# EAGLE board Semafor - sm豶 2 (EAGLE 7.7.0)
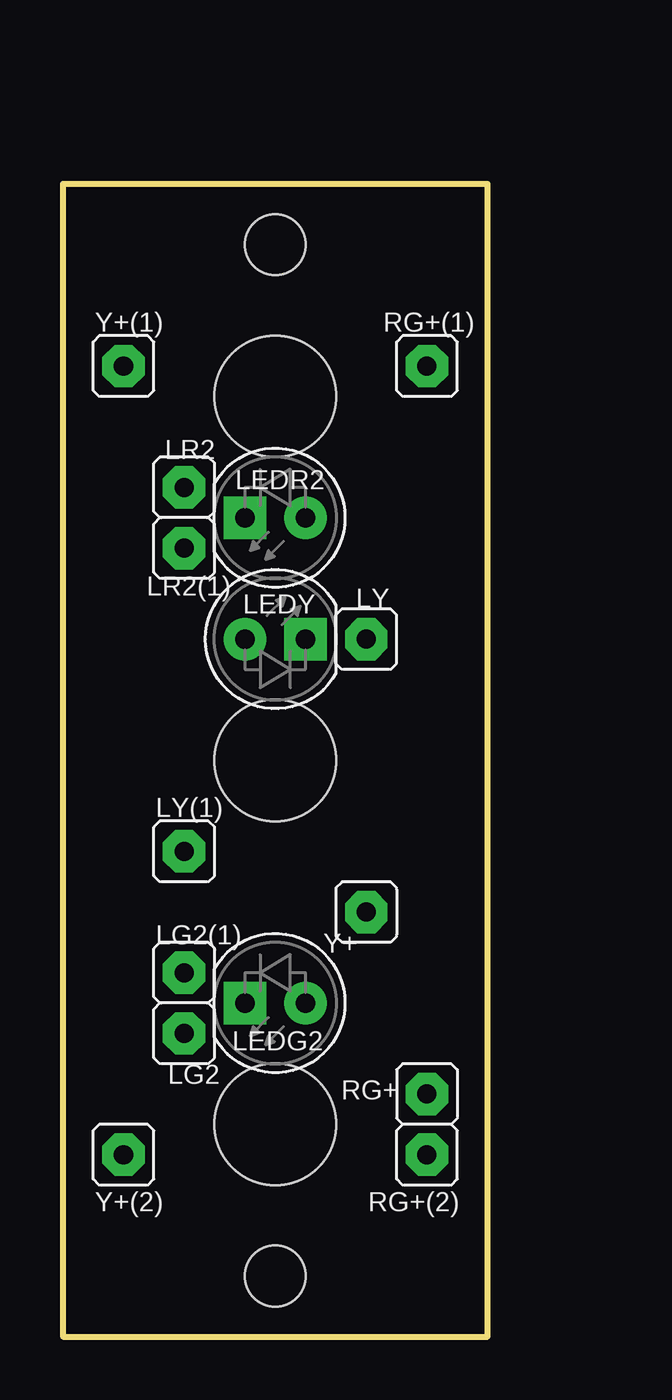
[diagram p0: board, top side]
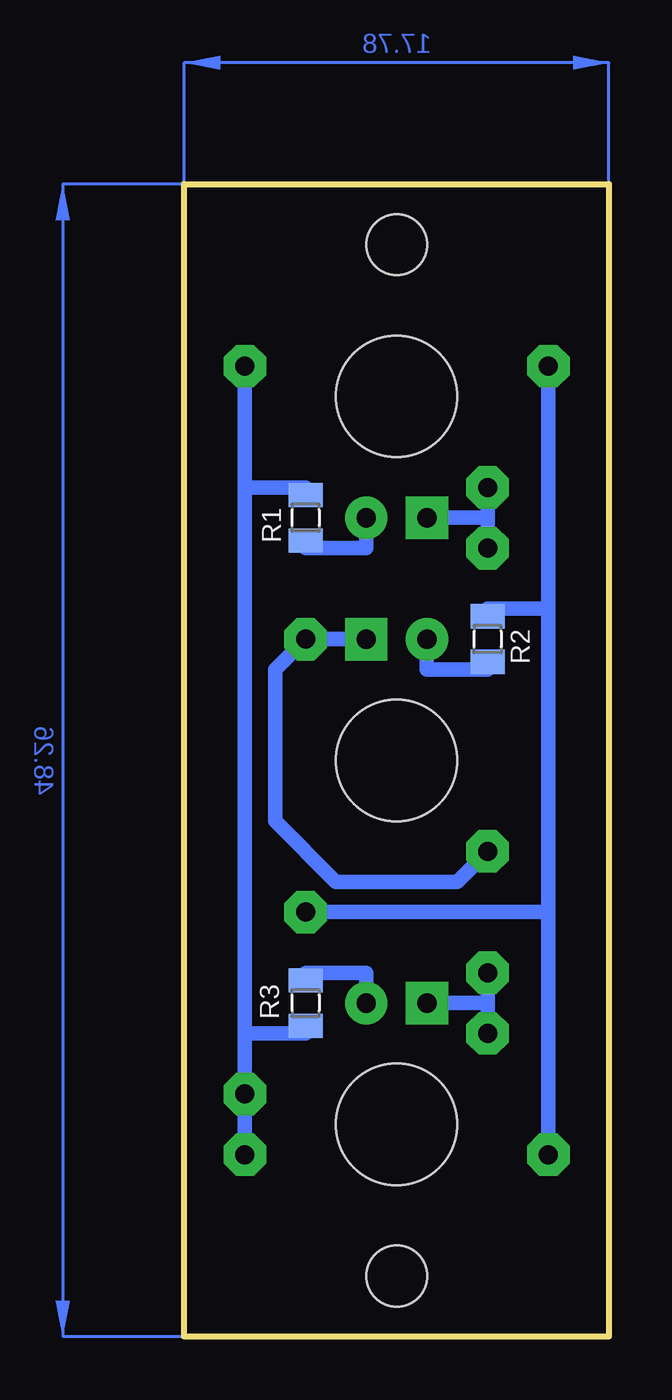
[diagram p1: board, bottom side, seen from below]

Size 17.78 x 48.26 mm. Coordinates in mm from the lower left corner, seen from the top.
Outline: 0,0 17.78,0 17.78,48.26 0,48.26 0,0
Copper layers (1*16): Top 0.035mm / dielectric 1.5mm / Bottom 0.035mm
Design rules "default": minimum track width 10mil, minimum drill 24mil, track to track 8mil, track to pad 8mil, pad to pad 8mil, via to via 8mil, smd to smd 8mil, copper to edge 40mil, drill to drill 8mil, minimum pad ring 10mil, minimum via ring 8mil, stop-mask expansion 4mil, vias tented up to drill 0mil, thermal gap 10mil
Holes 5.08 mm at 8.89,39.37 8.89,24.13 8.89,8.89
Holes 2.54 mm at 8.89,2.54 8.89,45.72

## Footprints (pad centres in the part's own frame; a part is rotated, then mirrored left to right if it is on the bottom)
LED_5 = drill 0.813 pad 1.778: A -1.27,0 | drill 0.813 pad 1.778 square: K 1.27,0
S1G1_JUM = drill 0.8 pad 1.778 octagon: 1 0,0
0805 = smd 1.016 x 1.422: 1 -0.953,0; 2 0.953,0

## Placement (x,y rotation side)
LEDG2  [LED_5]  8.89,13.97 180 top
LEDR2  [LED_5]  8.89,34.29 180 top
LEDY  [LED_5]  8.89,29.21 0 top
LG2  [S1G1_JUM]  5.08,12.7 270 top
LG2(1)  [S1G1_JUM]  5.08,15.24 270 top
LR2  [S1G1_JUM]  5.08,35.56 270 top
LR2(1)  [S1G1_JUM]  5.08,33.02 270 top
LY  [S1G1_JUM]  12.7,29.21 270 top
LY(1)  [S1G1_JUM]  5.08,20.32 270 top
R1  680R  [0805]  12.7,34.29 270 bottom
R2  680R  [0805]  5.08,29.21 270 bottom
R3  680R  [0805]  12.7,13.97 90 bottom
RG+  [S1G1_JUM]  15.24,10.16 0 top
RG+(1)  [S1G1_JUM]  15.24,40.64 270 top
RG+(2)  [S1G1_JUM]  15.24,7.62 270 top
Y+  [S1G1_JUM]  12.7,17.78 0 top
Y+(1)  [S1G1_JUM]  2.54,40.64 270 top
Y+(2)  [S1G1_JUM]  2.54,7.62 270 top

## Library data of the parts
LEDG2 LEDR2 LEDY R1-R3 = 1pomocná
LG2 LG2(1) LR2 LR2(1) LY LY(1) RG+ RG+(1) RG+(2) Y+ Y+(1) Y+(2) = #PaJa_konektory

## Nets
N$8: LEDR2.A R1.2
N$10: LEDR2.K LR2(1).1 LR2.1
N$11: LEDY.A R2.2
N$12: R2.1 Y+(1).1 Y+(2).1 Y+.1
N$13: LEDY.K LY(1).1 LY.1
N$14: LEDG2.A R3.2
N$15: LEDG2.K LG2(1).1 LG2.1
N$16: R1.1 R3.1 RG+(1).1 RG+(2).1 RG+.1

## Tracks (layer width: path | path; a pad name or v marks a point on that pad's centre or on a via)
N$8
  Bottom 0.61: LEDR2.A 10.16,33.02 12.7,33.02 R1.2
N$10
  Bottom 0.61: LEDR2.K 5.08,34.29 | 5.08,34.29 LR2(1).1 | LR2.1 5.08,34.29
N$11
  Bottom 0.61: LEDY.A 7.62,27.94 5.08,27.94 R2.2
N$12
  Bottom 0.61: 2.54,30.48 Y+(1).1 | R2.1 5.08,30.48 2.54,30.48 | 2.54,30.48 2.54,17.78 | 2.54,17.78 Y+(2).1 | Y+.1 2.54,17.78
N$13
  Bottom 0.61: LEDY.K LY.1 13.97,27.94 13.97,21.59 11.43,19.05 6.35,19.05 LY(1).1
N$14
  Bottom 0.61: LEDG2.A 10.16,15.24 12.7,15.24 R3.2
N$15
  Bottom 0.61: LEDG2.K 5.08,13.97 | 5.08,13.97 LG2(1).1 | LG2.1 5.08,13.97
N$16
  Bottom 0.61: 15.24,12.7 RG+.1 RG+(2).1 | 15.24,12.7 15.24,35.56 | 15.24,35.56 RG+(1).1 | R1.1 12.7,35.56 15.24,35.56 | R3.1 12.7,12.7 15.24,12.7
(copper drawn outside any net)
  shapes: Bottom area x2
